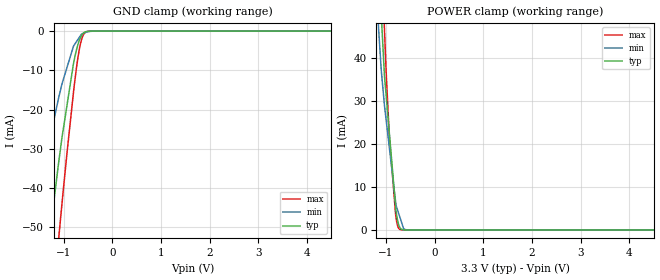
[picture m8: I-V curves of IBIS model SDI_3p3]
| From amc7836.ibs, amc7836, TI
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|   Model
[Model]   SDI_3p3
Model_type   Input
Vinl = 0.99
Vinh = 2.31
|   typ   min   max
C_comp   5.695pF   5.385pF   6.233pF
[Voltage Range]   3.3   3.29   3.31
[Temperature Range]   27   125   -40
[Power Clamp Reference]   3.3   3.29   3.31
[GND Clamp Reference]   0   0   0
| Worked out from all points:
|   GND clamp passes 1 mA (typ) near -0.62 V on its own axis
|   POWER clamp passes 1 mA (typ) near -0.73 V on its own axis
[GND Clamp]
|   Voltage   I(typ)   I(min)   I(max)
-3.3V     -293.4mA   -195.7mA   -362.8mA
-1.766V   -105.8mA   -61.2mA    -145mA
-1.606V   -87.25mA   -49.32mA   -122.4mA
-1.28V    -51.49mA   -27.36mA   -77.03mA
-1.092V   -32.68mA   -16.53mA   -51.73mA
-1.033V   -27.15mA   -13.47mA   -44.01mA
-933.9mV  -19.26mA   -9.447mA   -31.56mA
-798.2mV  -8.433mA   -3.932mA   -15.83mA
-735.9mV  -4.854mA   -2.709mA   -9.493mA
-646.8mV  -1.481mA   -1.052mA   -2.922mA
-557.7mV  -236.7uA   -341.8uA   -401.9uA
6.6V      0A         0A         0A
[POWER Clamp]
|   Voltage   I(typ)   I(min)   I(max)
-3.3V     807.6mA    663.4mA    932mA
-1.28V    102mA      69.51mA    132.3mA
-1.092V   48.63mA    36.26mA    65.28mA
-1.033V   35.78mA    28.88mA    46.55mA
-993.3mV  30.53mA    25.02mA    35.49mA
-933.9mV  22.64mA    19.23mA    21.98mA
-803.8mV  5.372mA    6.532mA    3.576mA
-765.6mV  2.369mA    4.68mA     1.093mA
-706.2mV  402.6uA    2.627mA    79.14uA
-636.9mV  31.35uA    230.3uA    2.758uA
-537.9mV  622.9nA    14.62uA    0A
6.6V      0A         0A         0A
